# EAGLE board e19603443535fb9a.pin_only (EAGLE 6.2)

Size 27.94 x 17.14 mm. Coordinates in mm from the lower left corner, seen from the top.
Outline: 27.94,14.61 27.94,2.54 arc-90 25.4,0 2.54,0 arc-90 0,2.54 0,14.61 arc-90 2.54,17.14 25.4,17.14 arc-90 27.94,14.61
Copper layers (1*16): Top 0.035mm / dielectric 1.5mm / Bottom 0.035mm
Design rules: minimum track width 8mil, minimum drill 0.4mm, track to track 8mil, track to pad 8mil, pad to pad 8mil, via to via 8mil, smd to smd 8mil, copper to edge 20mil, drill to drill 8mil, minimum pad ring 8mil, minimum via ring 10mil, stop-mask expansion 3mil, vias tented up to drill 20mil, thermal gap 8mil

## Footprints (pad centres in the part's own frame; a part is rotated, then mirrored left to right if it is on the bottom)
0805 = smd 1.3 x 1.5: 1 -0.95,0; 2 0.95,0
FIDUCIAL_1MM = smd 1 x 1: 1 0,0
1X10_ROUND70 = drill 1 pad 1.778: 1 -11.43,0; 2 -8.89,0; 3 -6.35,0; 4 -3.81,0; 5 -1.27,0; 6 1.27,0; 7 3.81,0; 8 6.35,0; 9 8.89,0; 10 11.43,0
MSOP10 = smd 0.25 x 1: 1 -1,-2.113; 2 -0.5,-2.113; 3 0,-2.113; 4 0.5,-2.113; 5 1,-2.113; 6 1,2.113; 7 0.5,2.113; 8 0,2.113; 9 -0.5,2.113; 10 -1,2.113
MOUNTINGHOLE_2.5_PLATED = drill 2.5 pad 3.2: P$1 0,0

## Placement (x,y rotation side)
C1  1µF  [0805]  21.59,12.32 0 top
C2  1µF  [0805]  3.81,7.24 0 top
FB1  MMZ2012Y152B  [0805]  2.79,10.29 90 top
FB2  MMZ2012Y152B  [0805]  5.08,10.29 90 top
FID1  FIDUCIAL""  [FIDUCIAL_1MM]  26.42,5.97 180 top
FID2  FIDUCIAL""  [FIDUCIAL_1MM]  17.53,13.72 180 top
JP1  [1X10_ROUND70]  13.97,1.91 180 top
R1  10K  [0805]  7.62,10.29 270 top
R2  10K  [0805]  10.16,10.29 270 top
R3  10K  [0805]  12.7,10.29 90 top
R4  10K  [0805]  15.24,10.29 270 top
U1  ADS1115IDGST  [MSOP10]  21.59,9.53 270 top
U$13  MOUNTINGHOLE2.5  [MOUNTINGHOLE_2.5_PLATED]  25.4,14.61 180 top
U$14  MOUNTINGHOLE2.5  [MOUNTINGHOLE_2.5_PLATED]  2.54,14.61 180 top
U$15  [ADAFRUIT_TEXT_20MM]  23.88,5.46 0 bottom
U$16  [ADAFRUIT_2.5MM]  16.51,6.22 0 top

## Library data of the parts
C1 C2 FB1 FB2 FID1 FID2 JP1 R1-R4 U1 U$13-U$16 = microbuilder

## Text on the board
tPlace: 16Bit I2C ADC+PGA | ADS1115 | ADDR | ALRT | VDD | GND | SCL | SDA | A0 | A1 | A2 | A3
bPlace: Max AIN: VDD | VDD: 2.0-5.5V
